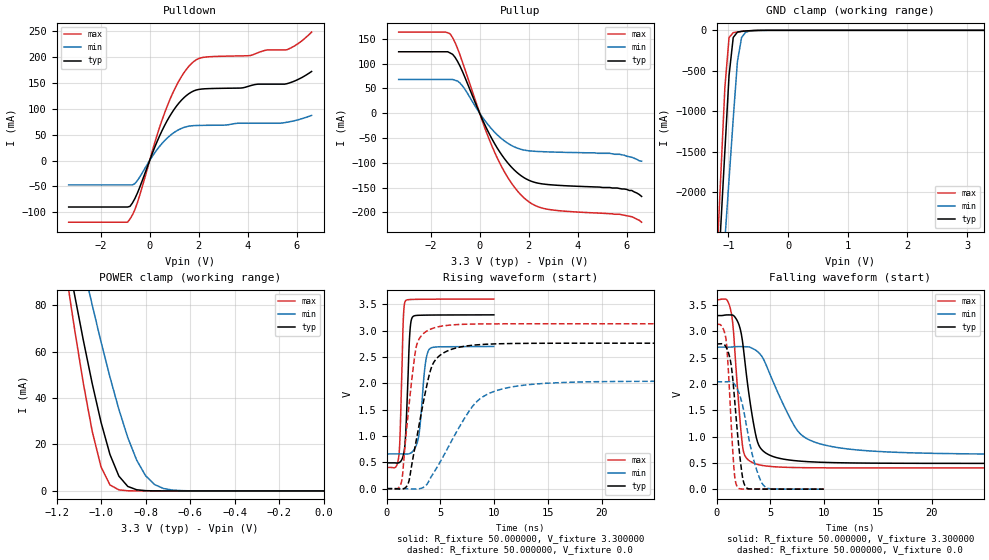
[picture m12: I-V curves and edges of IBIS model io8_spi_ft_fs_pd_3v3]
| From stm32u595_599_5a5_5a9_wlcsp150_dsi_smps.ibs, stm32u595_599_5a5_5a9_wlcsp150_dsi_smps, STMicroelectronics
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|   Model io8_spi_ft_fs_pd_3v3
[Model]  io8_spi_ft_fs_pd_3v3
Model_type I/O
Polarity   Non-Inverting
Enable   Active-Low
Vinl =   0.990000V
Vinh =   2.310000V
Vmeas =  1.650000V
Cref =   50.000000pF
Rref =   100.000000M
Vref =   0.0V
C_comp   3.495300pF   3.468500pF   3.534700pF
[Temperature Range]   25.000000   0.140000k   -40.000000
[Pullup Reference]   3.300000V   2.700000V   3.600000V
[Pulldown Reference]   0.0V   0.0V   0.0V
[POWER Clamp Reference]   3.300000V   2.700000V   3.600000V
[GND Clamp Reference]   0.0V   0.0V   0.0V
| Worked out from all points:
|   slope of the pulldown table from 0 to 0.495 V, typ, clamps not added: 8.73 ohm
|   slope of the pullup table from 0 to 0.495 V, typ, clamps not added: 9.64 ohm
|   GND clamp passes 1 mA (typ) near -0.50 V on its own axis
|   POWER clamp passes 1 mA (typ) near -0.85 V on its own axis
|   rising waveform, R_fixture 50.000000, V_fixture 3.300000: 20-80 % time 323ps typ, 519ps min, 256ps max; typ from 0.49 V to 3.3 V
|   rising waveform, R_fixture 50.000000, V_fixture 0.0: 20-80 % time 1.6ns typ, 3.59ns min, 973ps max; typ from 0 V to 2.76 V
|   falling waveform, R_fixture 50.000000, V_fixture 3.300000: 20-80 % time 1.16ns typ, 2.96ns min, 707ps max; typ from 3.3 V to 0.49 V
|   falling waveform, R_fixture 50.000000, V_fixture 0.0: 20-80 % time 757ps typ, 1.29ns min, 517ps max; typ from 2.76 V to 0 V
[Pulldown]
|Voltage   I(typ)   I(min)   I(max)
-3.3V     -89.72mA   -47.06mA   -119mA
-900mV    -89.72mA   -47.06mA   -119mA
-700mV    -81.75mA   -47.06mA   -104.8mA
-500mV    -62.92mA   -38.71mA   -81.44mA
300mV     36.2mA     21.01mA    48.7mA
800mV     84.06mA    46.96mA    114.8mA
1.3V      116.7mA    62.08mA    162.3mA
1.8V      134.4mA    67.38mA    191.2mA
2.2V      138.3mA    67.91mA    199.2mA
4.1V      144.4mA    71.97mA    202.7mA
5.6V      148.4mA    73.93mA    213.9mA
6.6V      171.9mA    87.1mA     247.9mA
[Pullup]
|Voltage   I(typ)   I(min)   I(max)
-3.3V     123.9mA    67.96mA    163.6mA
-1.2V     121.4mA    67.96mA    159.8mA
-1V       112.5mA    66.34mA    142.3mA
-700mV    83.98mA    54.94mA    103mA
200mV     -22.26mA   -14.13mA   -28.39mA
700mV     -69mA      -42.82mA   -88.5mA
1.3V      -109.1mA   -65.19mA   -141.4mA
1.9V      -132.8mA   -75.24mA   -174.9mA
2.7V      -143.6mA   -78mA      -193.2mA
5.6V      -151mA     -83mA      -204mA
6.2V      -156mA     -89mA      -209mA
6.6V      -168mA     -97mA      -220mA
[GND_clamp]
|Voltage   I(typ)   I(min)   I(max)
-3.3V     -9.098A    -9.372A    -9.671A
-1.2V     -3.386A    -4.091A    -2.933A
-1.13V    -2.437A    -3.34A     -1.815A
-1.06V    -1.49A     -2.588A    -705.6mA
-990mV    -555.7mA   -1.839A    -89.05mA
-920mV    -88.14mA   -1.093A    -28.79mA
-850mV    -22.36mA   -387.4mA   -19.86mA
-780mV    -12.13mA   -88.01mA   -13.89mA
-710mV    -7.72mA    -22.53mA   -8.86mA
-640mV    -4.556mA   -7.872mA   -4.884mA
-360mV    -39.69uA   -179.8uA   -19.45uA
3.28V     83.52uA    56.87uA    102.4uA
[POWER_clamp]
|Voltage   I(typ)   I(min)   I(max)
-3.28V    1.355A     1.167A     1.664A
-1.16V    105.7mA    131.6mA    95.69mA
-1.12V    84.97mA    114mA      70.27mA
-1.08V    65.05mA    96.83mA    46.54mA
-1.04V    46.34mA    80.15mA    25.76mA
-1V       29.51mA    64.13mA    10.3mA
-960mV    15.69mA    48.99mA    2.571mA
-920mV    6.373mA    35.1mA     455.6uA
-840mV    490.7uA    13.24mA    11.36uA
-760mV    27.33uA    2.767mA    279.3nA
-640mV    348nA      134.1uA    17.46nA
0V        0A         19.95nA    0A
[Ramp]
| variable   typ   min   max
dV/dt_r  1.65672/1.59920n   1.22424/3.58483n   1.87812/0.97272n
dV/dt_f  1.68575/1.16024n   1.22387/2.95616n   1.91751/0.70477n
R_load = 50.000000
[Rising Waveform]
R_fixture= 50.000000
V_fixture= 3.300000
V_fixture_min= 2.700000
V_fixture_max= 3.600000
|time   V(typ)   V(min)   V(max)
0s        489.8mV    659.6mV    403.5mV
1.141ns   491.1mV    659.6mV    616.8mV
1.562ns   633.6mV    659.3mV    3.225V
1.762ns   975.8mV    658.2mV    3.565V
2.142ns   2.883V     665.2mV    3.59V
2.402ns   3.254V     700.2mV    3.592V
3.023ns   3.291V     1.041V     3.595V
3.564ns   3.294V     2.301V     3.596V
3.944ns   3.295V     2.639V     3.596V
9.97ns    3.299V     2.699V     3.599V
[Rising Waveform]
R_fixture= 50.000000
V_fixture= 0.0
V_fixture_min= 0.0
V_fixture_max= 0.0
|time   V(typ)   V(min)   V(max)
0s        4.19uV     5.101uV    1.465uV
1.401ns   -9.732mV   80.94uV    132.9mV
2.002ns   91.11mV    -2.094mV   1.407V
2.503ns   633.8mV    -7.865mV   2.333V
2.803ns   961.8mV    -7.306mV   2.728V
3.904ns   2.107V     132.7mV    3.01V
4.505ns   2.434V     342.7mV    3.058V
8.208ns   2.727V     1.615V     3.125V
11.41ns   2.755V     1.923V     3.13V
49.85ns   2.761V     2.04V      3.13V
[Falling Waveform]
R_fixture= 50.000000
V_fixture= 3.300000
V_fixture_min= 2.700000
V_fixture_max= 3.600000
|time   V(typ)   V(min)   V(max)
0s        3.299V     2.699V     3.599V
1.301ns   3.311V     2.7V       3.42V
1.602ns   3.296V     2.705V     2.933V
2.102ns   3.115V     2.709V     1.502V
2.603ns   2.487V     2.708V     650.1mV
3.704ns   974.5mV    2.633V     476.8mV
4.705ns   670.8mV    2.313V     438.1mV
7.508ns   537.6mV    1.116V     410.4mV
10.51ns   506.4mV    817.6mV    405.1mV
49.85ns   489.8mV    659.6mV    403.5mV
[Falling Waveform]
R_fixture= 50.000000
V_fixture= 0.0
V_fixture_min= 0.0
V_fixture_max= 0.0
|time   V(typ)   V(min)   V(max)
0s        2.761V     2.04V      3.13V
880.9ps   2.702V     2.041V     2.847V
1.301ns   2.43V      2.043V     1.482V
1.622ns   1.843V     2.006V     388.4mV
1.942ns   1.074V     1.9V       40.89mV
2.382ns   271mV      1.625V     3.287mV
2.623ns   73.54mV    1.389V     2.378mV
3.383ns   3.04mV     610.3mV    1.306mV
4.324ns   1.388mV    83.53mV    829uV
9.97ns    4.19uV     5.101uV    1.465uV
